(* Logix 5000 AddOnInstructionDefinition export AMCI_MA_SV_Linear_Follower; software revision 31.02 *)

TYPE AMCI_Motion_Axis_Input_Data :
STRUCT
   Moving_CW : BOOL;
   Moving_CCW : BOOL;
   In_Hold_State : BOOL;
   Stopped : BOOL;
   At_Home : BOOL;
   Accelerating : BOOL;
   Decelerating : BOOL;
   Move_Complete : BOOL;
   Status_Word_0_Bit_8 : BOOL;
   Status_Word_0_Bit_9 : BOOL;
   Position_Invalid : BOOL;
   Input_Error : BOOL;
   Command_Error : BOOL;
   Configuration_Error : BOOL;
   Module_OK : BOOL;
   Mode_Flag : BOOL;
   IN1_Active : BOOL;
   IN2_Active : BOOL;
   IN3_Active : BOOL;
   IN4_Active : BOOL;
   Status_Word_1_Bit_4 : BOOL;
   Status_Word_1_Bit_5 : BOOL;
   Connection_Was_Lost : BOOL;
   Driver_Fault : BOOL;
   Status_Word_1_Bit_8 : BOOL;
   Invalid_Jog_Change : BOOL;
   Status_Word_1_Bit_10 : BOOL;
   Heartbeat_Bit : BOOL;
   Status_Word_1_Bit_12 : BOOL;
   Status_Word_1_Bit_13 : BOOL;
   Stall_Detected : BOOL;
   Drive_Is_Enabled : BOOL;
   Motor_Position : DINT;
   Encoder_Position : DINT;
   Trapped_Encoder_Position : DINT;
   Input_Word_8 : INT;
   Input_Word_9 : INT;
END_STRUCT
END_TYPE

TYPE AMCI_Motion_Axis_Output_Data :
STRUCT
   Control_Word_0 : INT;
   Control_Word_1 : INT;
   Position_or_Distance : DINT;
   Programmed_Speed : DINT;
   Acceleration : INT;
   Deceleration : INT;
   Output_Word_8 : INT;
   Output_Word_9 : INT;
END_STRUCT
END_TYPE

ADD_ON_INSTRUCTION AMCI_MA_SV_Linear_Follower   (* revision 1.1, vendor AMCI, ExecuteEnableInFalse *)
// Only for SVXXXE2 motion devices.
// Revision note:
// Version 1.1:  Corrected mistake in the text on the Help Tab.
// Help:
// MOTION AXIS SV CIRCULAR FOLLOWER
// These AOIs will only work with the SV motion devices.  The SMD and SD  motion devices have their own follower AOIs.
// AXIS INPUT DATA:  Input data from AMCI motion device.   Uses the AMCI_Motion_Axis_Input_Data User Defined Data Type.
// AXIS OUTPUT DATA; Output data from the AOI to the AMCI motion device.   Uses the AMCI_Motion_Axis_Output_Data User Defined Data Type.
// FOLLOWER POSITION: REAL DATA TYPE position directly from the motion axis.
// FOLLOWER VELOCITY: REAL DATA TYPE velocity directly from the motion axis.
// FOLLOWER ACCELERATION: REAL DATA TYPE acceleration directly from the motion axis.
// RAMP ACCELERATION: An actual value or INT value used to transition from no motion to motion.   Once
//                                          motion is occurring, the follower acceleration will be used.  Range of 0 to 15,999.
// DECELERATION: An actual value or INT value used to transition from motion to no motion.   Range of 0 to
//                              15,999.
// EN (Enable) Set when rung is true, Reset when rung is false
// DN (Done) Set when command is sent to the motion device.  Reset when the rung is false.
// ER (Error) Set when a command or input error failed to clear.  Reset when the rung is false.
// IP (In Process) Set when motion is occurring.   Reset when the rung goes false.
VAR_IN_OUT
   Axis_Input_Data : AMCI_Motion_Axis_Input_Data; {required}
   Axis_Output_Data : AMCI_Motion_Axis_Output_Data; {required}
END_VAR
VAR_INPUT
   Follower_Position : REAL; {required}
   Follower_Velocity : REAL; {required}
   Follower_Acceleration : REAL; {required}
   Ramp_Acceleration : INT; {required}
   Deceleration : INT; {required}
   Maximum_Move_Torque : INT;
END_VAR
VAR_OUTPUT
   EN : BOOL; {visible}
   ER : BOOL; {visible}
   DN : BOOL; {access Read Only, visible}
   IP : BOOL; {access Read Only, visible}
END_VAR
VAR
   command_data_block : INT[10];
        [0]   // Command Bits MSW
        [1]   // Command Bits LSW
        [2]   // Upper Target Position
        [3]   // Lower Target Position
        [4]   // Upper Programmed Speed
        [5]   // Lower Programmed Speed
   axis_follower_position : DINT;
   axis_follower_velocity : DINT;
END_VAR

ROUTINE EnableInFalse   (* ladder *)
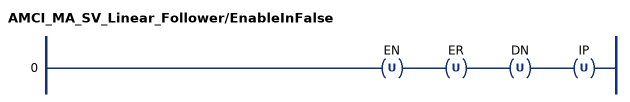
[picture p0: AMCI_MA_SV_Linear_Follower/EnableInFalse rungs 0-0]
   0: OTU(EN)OTU(ER)OTU(DN)OTU(IP);
END_ROUTINE

ROUTINE Logic   (* ladder *)
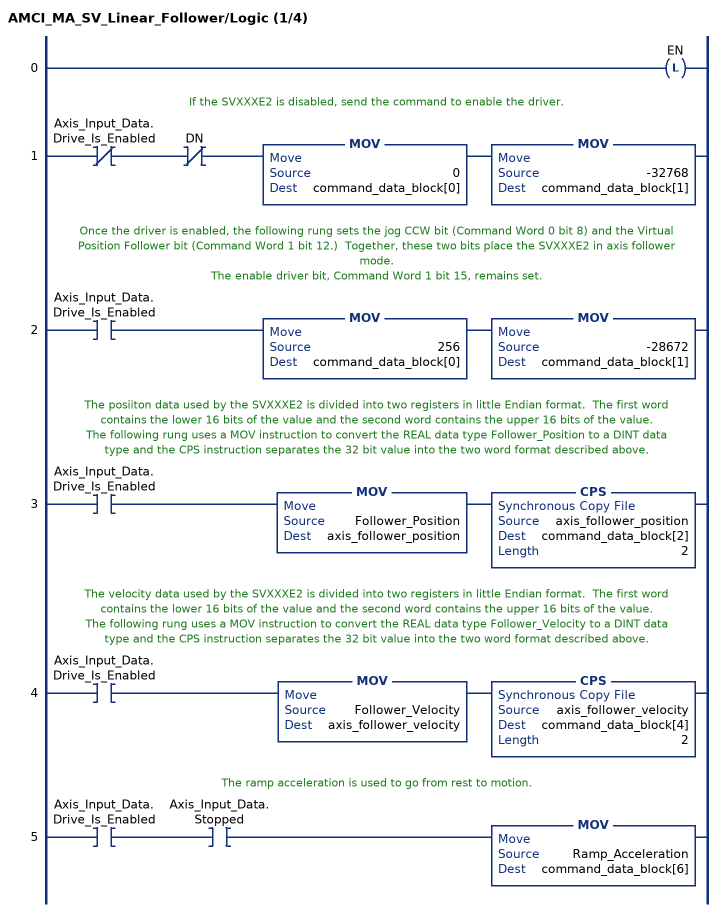
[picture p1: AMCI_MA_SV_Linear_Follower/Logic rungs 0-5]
   0: OTL(EN);
   // If the SVXXXE2 is disabled, send the command to enable the driver.
   1: XIO(Axis_Input_Data.Drive_Is_Enabled)XIO(DN)MOV(0,command_data_block[0])MOV(-32768,command_data_block[1]);
   // Once the driver is enabled, the following rung sets the jog CCW bit (Command Word 0 bit 8) and the Virtual Position Follower bit (Command Word 1 bit 12.)  Together, these two bits place the SVXXXE2 in axis follower mode.
   // The enable driver bit, Command Word 1 bit 15, remains set.
   2: XIC(Axis_Input_Data.Drive_Is_Enabled)MOV(256,command_data_block[0])MOV(-28672,command_data_block[1]);
   // The posiiton data used by the SVXXXE2 is divided into two registers in little Endian format.  The first word contains the lower 16 bits of the value and the second word contains the upper 16 bits of the value.
   // The following rung uses a MOV instruction to convert the REAL data type Follower_Position to a DINT data type and the CPS instruction separates the 32 bit value into the two word format described above.
   3: XIC(Axis_Input_Data.Drive_Is_Enabled)MOV(Follower_Position,axis_follower_position)CPS(axis_follower_position,command_data_block[2],2);
   // The velocity data used by the SVXXXE2 is divided into two registers in little Endian format.  The first word contains the lower 16 bits of the value and the second word contains the upper 16 bits of the value.
   // The following rung uses a MOV instruction to convert the REAL data type Follower_Velocity to a DINT data type and the CPS instruction separates the 32 bit value into the two word format described above.
   4: XIC(Axis_Input_Data.Drive_Is_Enabled)MOV(Follower_Velocity,axis_follower_velocity)CPS(axis_follower_velocity,command_data_block[4],2);
   // The ramp acceleration is used to go from rest to motion.
   5: XIC(Axis_Input_Data.Drive_Is_Enabled)XIC(Axis_Input_Data.Stopped)MOV(Ramp_Acceleration,command_data_block[6]);
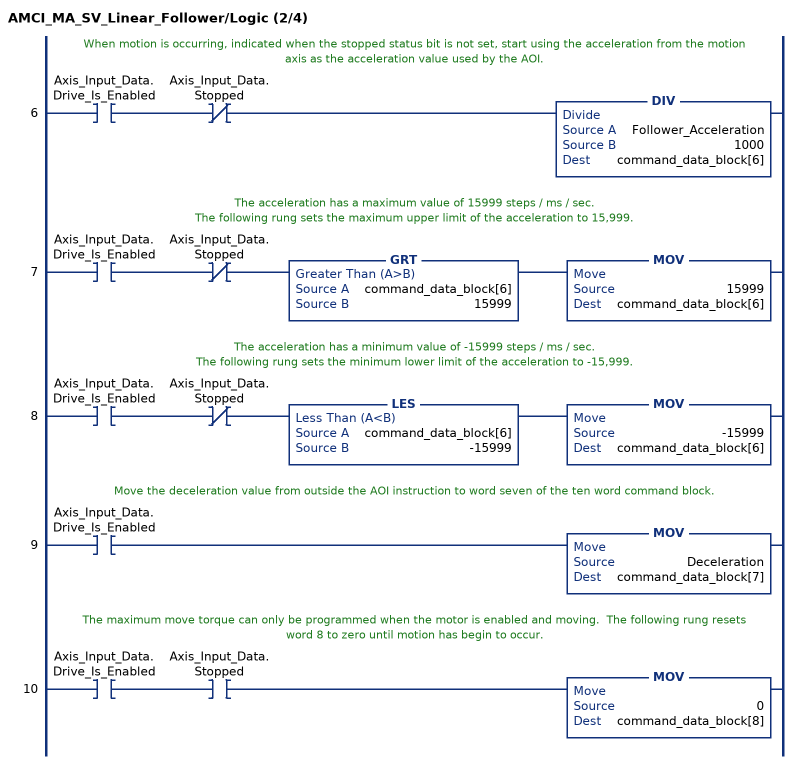
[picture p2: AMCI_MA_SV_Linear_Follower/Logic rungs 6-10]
   // When motion is occurring, indicated when the stopped status bit is not set, start using the acceleration from the motion axis as the acceleration value used by the AOI.
   6: XIC(Axis_Input_Data.Drive_Is_Enabled)XIO(Axis_Input_Data.Stopped)DIV(Follower_Acceleration,1000,command_data_block[6]);
   // The acceleration has a maximum value of 15999 steps / ms / sec.
   // The following rung sets the maximum upper limit of the acceleration to 15,999.
   7: XIC(Axis_Input_Data.Drive_Is_Enabled)XIO(Axis_Input_Data.Stopped)GRT(command_data_block[6],15999)MOV(15999,command_data_block[6]);
   // The acceleration has a minimum value of -15999 steps / ms / sec.
   // The following rung sets the minimum lower limit of the acceleration to -15,999.
   8: XIC(Axis_Input_Data.Drive_Is_Enabled)XIO(Axis_Input_Data.Stopped)LES(command_data_block[6],-15999)MOV(-15999,command_data_block[6]);
   // Move the deceleration value from outside the AOI instruction to word seven of the ten word command block.
   9: XIC(Axis_Input_Data.Drive_Is_Enabled)MOV(Deceleration,command_data_block[7]);
   // The maximum move torque can only be programmed when the motor is enabled and moving.  The following rung resets word 8 to zero until motion has begin to occur.
   10: XIC(Axis_Input_Data.Drive_Is_Enabled)XIC(Axis_Input_Data.Stopped)MOV(0,command_data_block[8]);
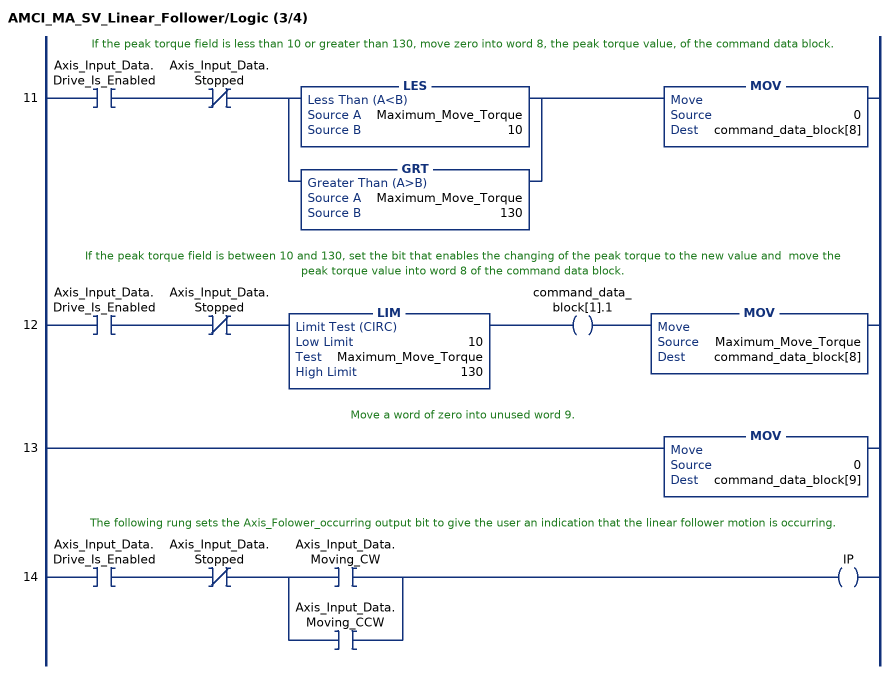
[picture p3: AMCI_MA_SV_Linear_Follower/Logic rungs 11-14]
   // If the peak torque field is less than 10 or greater than 130, move zero into word 8, the peak torque value, of the command data block.
   11: XIC(Axis_Input_Data.Drive_Is_Enabled)XIO(Axis_Input_Data.Stopped)[LES(Maximum_Move_Torque,10) ,GRT(Maximum_Move_Torque,130) ]MOV(0,command_data_block[8]);
   // If the peak torque field is between 10 and 130, set the bit that enables the changing of the peak torque to the new value and  move the peak torque value into word 8 of the command data block.
   12: XIC(Axis_Input_Data.Drive_Is_Enabled)XIO(Axis_Input_Data.Stopped)LIM(10,Maximum_Move_Torque,130)OTE(command_data_block[1].1)MOV(Maximum_Move_Torque,command_data_block[8]);
   // Move a word of zero into unused word 9.
   13: MOV(0,command_data_block[9]);
   // The following rung sets the Axis_Folower_occurring output bit to give the user an indication that the linear follower motion is occurring.
   14: XIC(Axis_Input_Data.Drive_Is_Enabled)XIO(Axis_Input_Data.Stopped)[XIC(Axis_Input_Data.Moving_CW) ,XIC(Axis_Input_Data.Moving_CCW) ]OTE(IP);
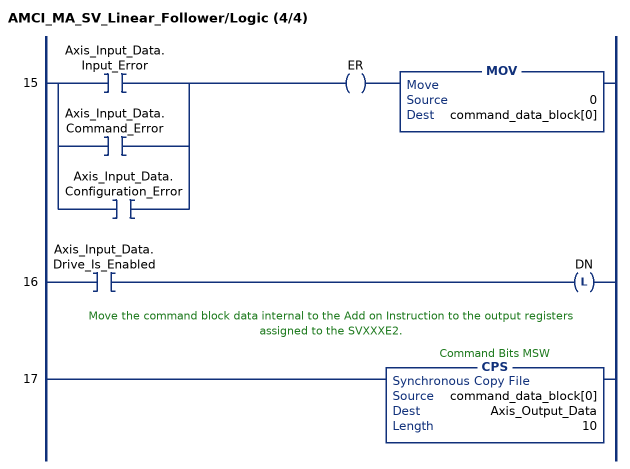
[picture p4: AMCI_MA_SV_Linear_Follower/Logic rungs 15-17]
   15: [XIC(Axis_Input_Data.Input_Error) ,XIC(Axis_Input_Data.Command_Error) ,XIC(Axis_Input_Data.Configuration_Error) ]OTE(ER)MOV(0,command_data_block[0]);
   16: XIC(Axis_Input_Data.Drive_Is_Enabled)OTL(DN);
   // Move the command block data internal to the Add on Instruction to the output registers assigned to the SVXXXE2.
   17: CPS(command_data_block[0],Axis_Output_Data,10);
END_ROUTINE
END_ADD_ON_INSTRUCTION
